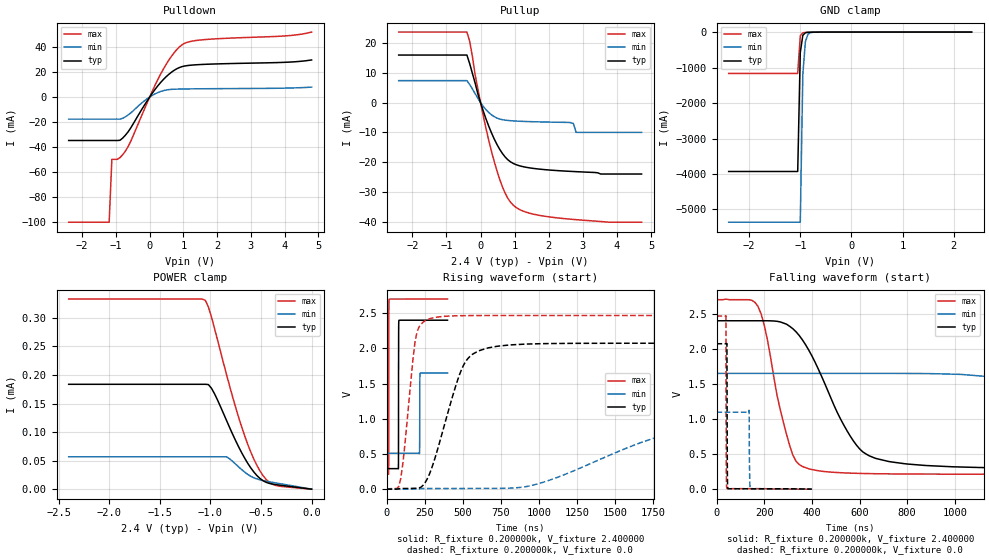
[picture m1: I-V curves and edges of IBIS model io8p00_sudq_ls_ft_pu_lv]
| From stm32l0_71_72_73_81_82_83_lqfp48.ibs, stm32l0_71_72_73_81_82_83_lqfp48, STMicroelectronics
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|   Model io8p00_sudq_ls_ft_pu_lv
[Model]  io8p00_sudq_ls_ft_pu_lv
Model_type I/O
Polarity   Non-Inverting
Enable   Active-Low
Vinl =   0.720000V
Vinh =   1.680000V
Vmeas =  1.200000V
Cref =   50.000000pF
Rref =   100.000000M
Vref =   0.0V
C_comp   2.317700pF   2.286600pF   2.332700pF
[Temperature Range]   25.000000   0.105000k   -40.000000
[Pullup Reference]   2.400000V   1.650000V   2.700000V
[Pulldown Reference]   0.0V   0.0V   0.0V
[POWER Clamp Reference]   2.400000V   1.650000V   2.700000V
[GND Clamp Reference]   0.0V   0.0V   0.0V
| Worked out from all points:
|   slope of the pulldown table from 0 to 0.36 V, typ, clamps not added: 28.4 ohm
|   slope of the pullup table from 0 to 0.36 V, typ, clamps not added: 32.2 ohm
|   GND clamp passes 1 mA (typ) near -0.65 V on its own axis
|   rising waveform, R_fixture 0.200000k, V_fixture 2.400000: 20-80 % time 634ps typ, 834ps min, 676ps max; typ from 0.292 V to 2.4 V
|   rising waveform, R_fixture 0.200000k, V_fixture 0.0: 20-80 % time 170ns typ, 825ns min, 67ns max; typ from 0.001 V to 2.07 V
|   falling waveform, R_fixture 0.200000k, V_fixture 2.400000: 20-80 % time 182ns typ, 736ns min, 90.7ns max; typ from 2.4 V to 0.292 V
|   falling waveform, R_fixture 0.200000k, V_fixture 0.0: 20-80 % time 1.15ns typ, 1.66ns min, 929ps max; typ from 2.07 V to 0.001 V
[Pulldown]
|Voltage   I(typ)   I(min)   I(max)
-2.4V     -34.71mA   -17.62mA   -100mA
-1.2V     -34.71mA   -17.62mA   -100mA
-1.12V    -34.71mA   -17.62mA   -49.77mA
-960mV    -34.71mA   -17.62mA   -49.77mA
-720mV    -30.52mA   -15.81mA   -43.24mA
-560mV    -24.66mA   -12.69mA   -35.31mA
-80mV     -3.3mA     -1.497mA   -4.982mA
320mV     11.47mA    4.39mA     18.08mA
640mV     19.72mA    6.139mA    32.34mA
960mV     24.33mA    6.432mA    41.77mA
1.52V     26.01mA    6.612mA    45.64mA
4.8V      29.64mA    7.944mA    51.92mA
[Pullup]
|Voltage   I(typ)   I(min)   I(max)
-2.4V     16.03mA    7.415mA    23.74mA
-400mV    16.03mA    7.415mA    23.74mA
-320mV    13.17mA    6.146mA    20.72mA
-160mV    6.616mA    3.072mA    9.467mA
80mV      -2.838mA   -1.261mA   -4.478mA
400mV     -12.2mA    -4.699mA   -19.76mA
720mV     -18.26mA   -5.869mA   -30.44mA
1.04V     -20.85mA   -6.184mA   -35.23mA
2.64V     -23.11mA   -6.7mA     -39.19mA
2.72V     -23.16mA   -7mA       -39.27mA
2.8V      -23.2mA    -10mA      -39.35mA
4.72V     -24mA      -10mA      -40.2mA
[GND_clamp]
|Voltage   I(typ)   I(min)   I(max)
-2.4V     -3.929A    -5.359A    -1.166A
-1.05V    -3.929A    -5.359A    -1.166A
-1V       -574.5mA   -5.359A    -109.1mA
-950mV    -90.02mA   -1.192A    -18.55mA
-900mV    -18.41mA   -269.7mA   -9.049mA
-850mV    -6.764mA   -63.59mA   -6.579mA
-800mV    -4.027mA   -16.66mA   -4.859mA
-650mV    -1.043mA   -1.218mA   -1.146mA
2.35V     0A         0A         0A
[POWER_clamp]
|Voltage   I(typ)   I(min)   I(max)
-2.4V     183.7uA    56.67uA    333uA
-1.05V    183.7uA    56.67uA    330.8uA
-1.02V    183.2uA    56.67uA    319.3uA
-960mV    167.4uA    56.67uA    282.2uA
-840mV    120.1uA    56.67uA    200.3uA
-750mV    84.75uA    43.78uA    142.9uA
-690mV    63.55uA    34.11uA    108.5uA
-600mV    37.04uA    22.44uA    64.62uA
-510mV    18.73uA    16.34uA    31.91uA
-450mV    12.06uA    14.02uA    17.25uA
-360mV    8.154uA    11.11uA    6.782uA
0V        0A         0A         0A
[Ramp]
| variable   typ   min   max
dV/dt_r  0.65095/0.30260u   0.19035/0.82157u   1.03793/0.14412u
dV/dt_f  0.75624/0.32406u   0.19656/0.85274u   1.13751/0.16141u
R_load = 50.000000
[Rising Waveform]
R_fixture= 0.200000k
V_fixture= 2.400000
V_fixture_min= 1.650000
V_fixture_max= 2.700000
|time   V(typ)   V(min)   V(max)
0s        291.9mV    510.4mV    213.7mV
14.01ns   291.9mV    510.4mV    220.6mV
15.22ns   291.9mV    510.4mV    2.501V
16.82ns   291.9mV    510.4mV    2.696V
77.68ns   290.1mV    510.4mV    2.7V
79.28ns   2.141V     510.4mV    2.7V
81.28ns   2.397V     510.4mV    2.7V
215.8ns   2.4V       502.4mV    2.7V
220.6ns   2.4V       1.647V     2.7V
400ns     2.4V       1.65V      2.7V
[Rising Waveform]
R_fixture= 0.200000k
V_fixture= 0.0
V_fixture_min= 0.0
V_fixture_max= 0.0
|time   V(typ)   V(min)   V(max)
0s        1.17mV     2.205mV    629.4uV
93.43ns   10.52mV    2.205mV    152.3mV
200.2ns   14.58mV    2.205mV    2.237V
280.3ns   208.8mV    9.997mV    2.418V
373.7ns   865.9mV    9.997mV    2.454V
547.2ns   1.886V     10.3mV     2.465V
920.9ns   2.061V     39.15mV    2.467V
1.949us   2.073V     850mV      2.467V
2.856us   2.073V     1.068V     2.467V
13.33us   2.073V     1.097V     2.467V
[Falling Waveform]
R_fixture= 0.200000k
V_fixture= 2.400000
V_fixture_min= 1.650000
V_fixture_max= 2.700000
|time   V(typ)   V(min)   V(max)
0s        2.4V       1.65V      2.7V
173.5ns   2.4V       1.65V      2.607V
320.3ns   2.286V     1.65V      485.2mV
533.9ns   914.2mV    1.65V      232.7mV
640.6ns   475.8mV    1.65V      222.3mV
867.5ns   340.4mV    1.648V     215.5mV
1.361us   298.4mV    1.498V     213.7mV
2.216us   292.2mV    727.7mV    213.7mV
3.083us   291.9mV    548.2mV    213.7mV
13.33us   291.9mV    510.4mV    213.7mV
[Falling Waveform]
R_fixture= 0.200000k
V_fixture= 0.0
V_fixture_min= 0.0
V_fixture_max= 0.0
|time   V(typ)   V(min)   V(max)
0s        2.073V     1.097V     2.467V
39.24ns   2.073V     1.097V     2.471V
40.84ns   2.073V     1.097V     356.7mV
43.24ns   2.076V     1.097V     12.25mV
45.25ns   350.5mV    1.097V     8.538mV
48.05ns   9.207mV    1.097V     8.435mV
136.5ns   6.328mV    1.123V     8.393mV
138.9ns   6.328mV    202mV      8.394mV
142.5ns   6.328mV    6.123mV    8.394mV
400ns     1.17mV     2.205mV    629.4uV
